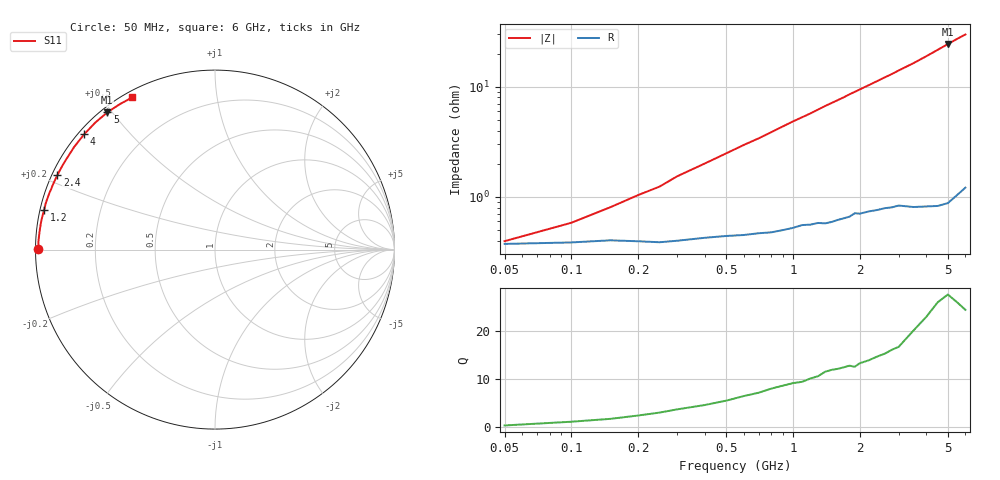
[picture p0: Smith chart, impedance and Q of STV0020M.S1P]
! SIEMENS Discrete & RF Semiconductors
! BA892
! Si PIN Diode in SCD-80
! IF = 20 mA
! S-Parameters:  September  1997
# GHz  S  MA  R  50
!  f  S11
! GHz  MAG  ANG
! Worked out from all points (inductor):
!   34 points, 50 MHz to 6 GHz, reference 50 ohm
!   read as one part to ground: L = 782 pH near 250 MHz
!   highest Q = 26.1 at 5 GHz (marker M1), where L = 774 pH
!   S11 on the Smith chart (normalised r, x): 50 MHz: 0.01, +0.00; 1.2 GHz: 0.01, +0.11; 2.4 GHz: 0.02, +0.22; 4 GHz: 0.02, +0.38; 5 GHz: 0.02, +0.49; 6 GHz: 0.02, +0.59
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0.05  0.9851 179.7
0.1  0.9847 179.0
0.15  0.984 178.4
0.2  0.9843 177.8
0.25  0.9846 177.3
0.3  0.9841 176.6
0.6  0.9822 173.3
0.7  0.9815 172.3
0.8  0.9812 171.2
1  0.9794 169.0
1.2  0.9781 167.0
1.4  0.9776 164.8
1.6  0.976 162.8
1.7  0.9753 161.8
1.8  0.9746 160.7
1.9  0.9728 159.7
2  0.9731 158.7
2.2  0.9721 156.7
2.4  0.9714 154.7
2.6  0.9706 152.7
2.8  0.9703 150.8
3  0.9695 148.7
3.5  0.9711 143.8
4  0.9717 138.6
4.5  0.9725 133.3
5  0.972 128.1
5.5  0.9684 123.1
6  0.9647 118.5
